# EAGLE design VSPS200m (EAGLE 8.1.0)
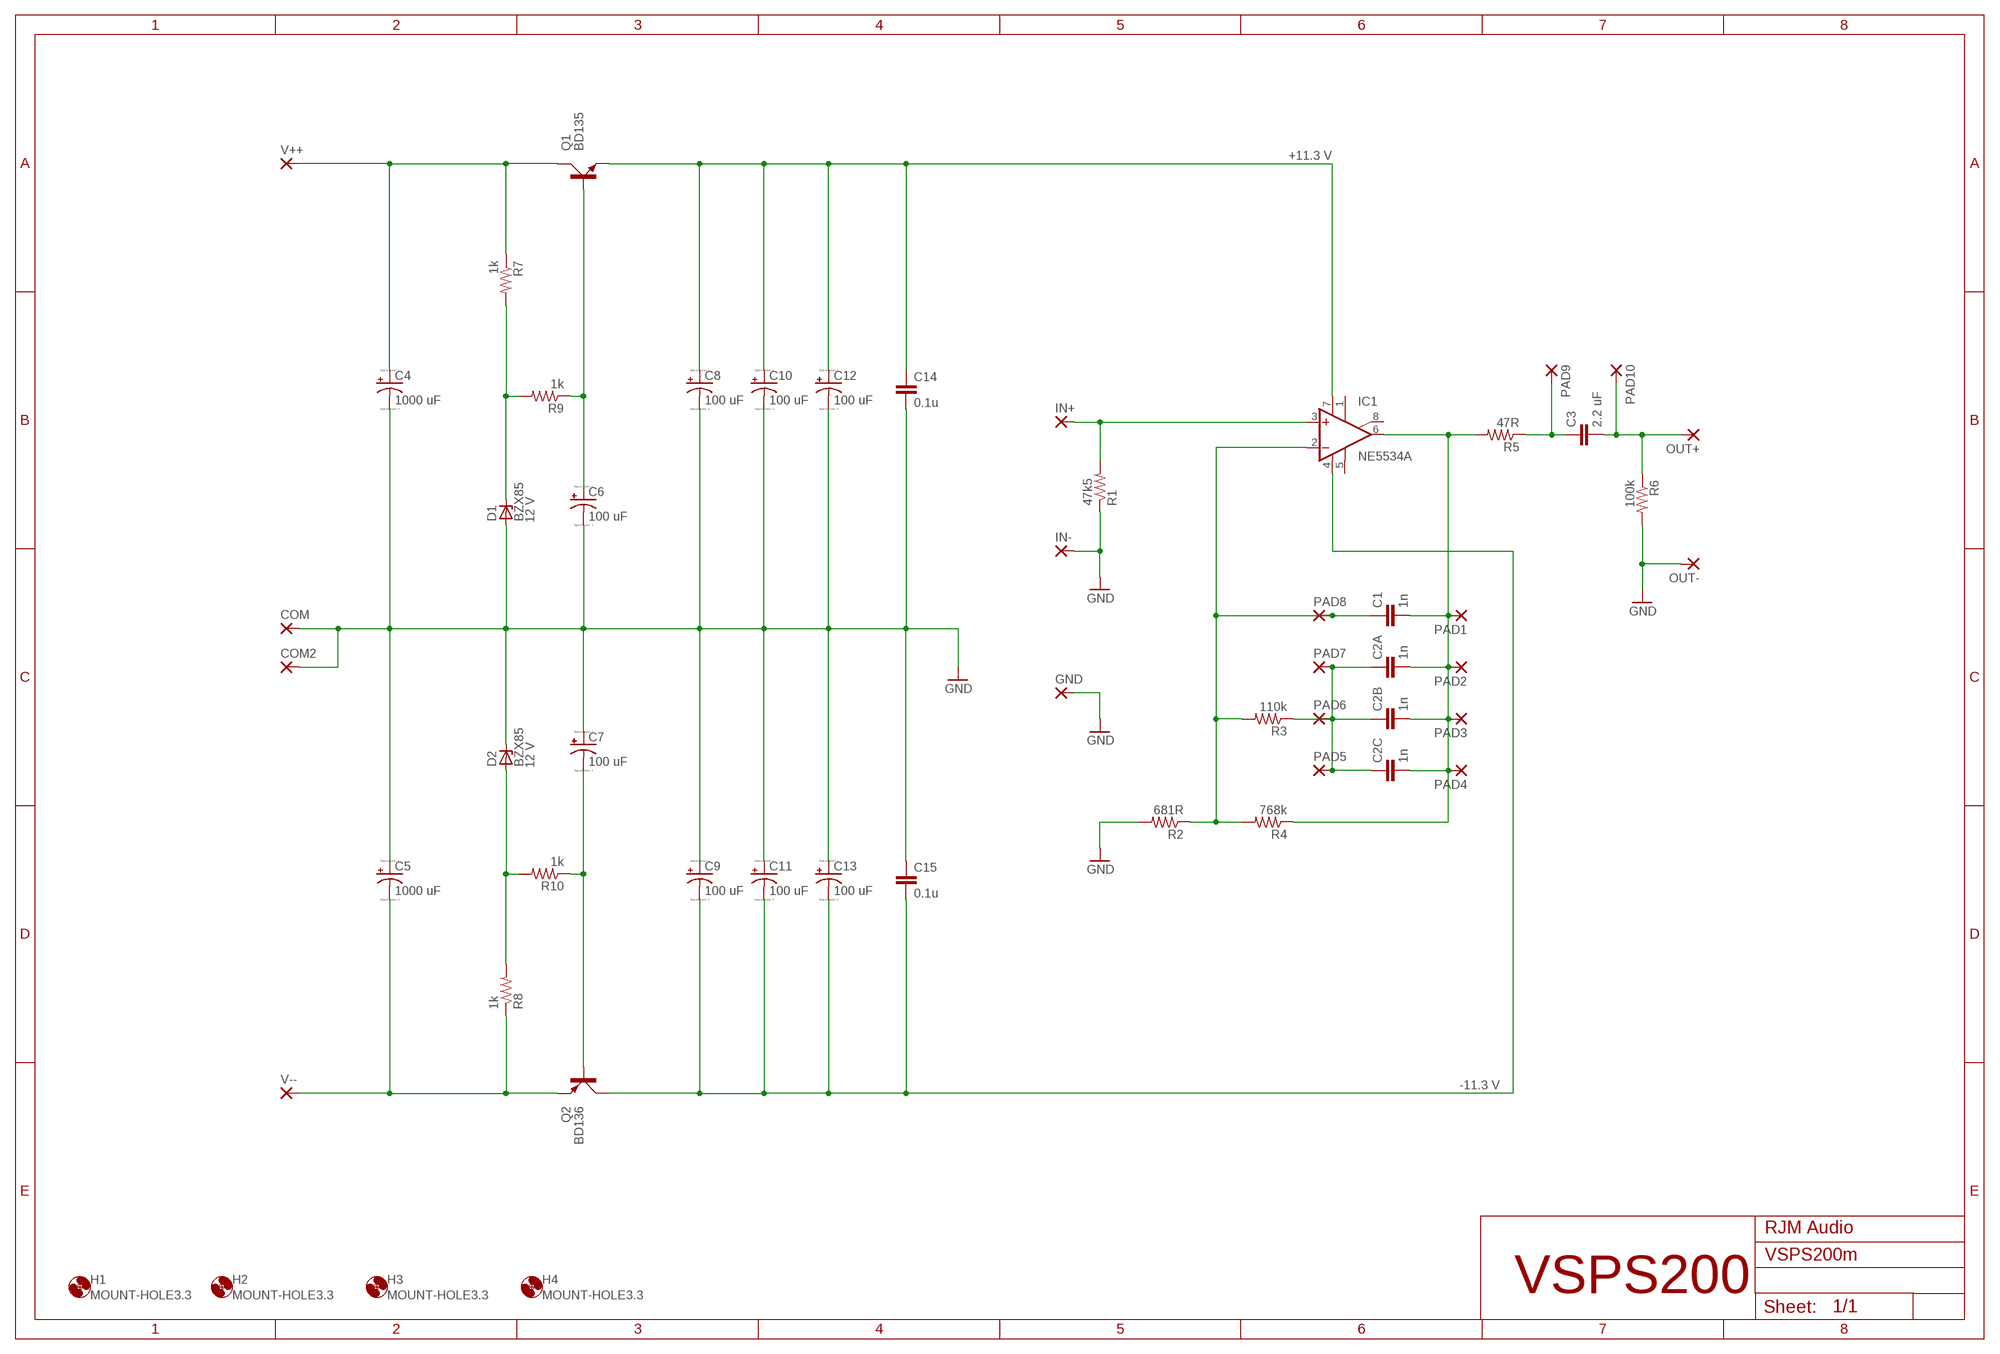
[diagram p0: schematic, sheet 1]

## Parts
C1  1n  C-EU050-045X075  [C050-045X075]
C2A  1n  C-EU050-045X075  [C050-045X075]
C2B  1n  C-EU050-045X075  [C050-045X075]
C2C  1n  C-EU050-045X075  [C050-045X075]
C3  2.2 uF  C-EU375-155X418  [C375-155X418]
C4  1000 uF  CPOL-USE5-10.5  [E5-10,5]
C5  1000 uF  CPOL-USE5-10.5  [E5-10,5]
C6  100 uF  CPOL-USE2.5-6  [E2,5-6]
C7  100 uF  CPOL-USE2.5-6  [E2,5-6]
C8  100 uF  CPOL-USE2.5-6  [E2,5-6]
C9  100 uF  CPOL-USE2.5-6  [E2,5-6]
C10  100 uF  CPOL-USE2.5-6  [E2,5-6]
C11  100 uF  CPOL-USE2.5-6  [E2,5-6]
C12  100 uF  CPOL-USE2.5-6  [E2,5-6]
C13  100 uF  CPOL-USE2.5-6  [E2,5-6]
C14  0.1u  C-EU050-024X044  [C050-024X044]
C15  0.1u  C-EU050-024X044  [C050-024X044]
COM  3,17/1,3  [3,17/1,3]
COM2  3,17/1,3  [3,17/1,3]
D1  BZX85  [DO41Z10]
D2  BZX85  [DO41Z10]
GND  3,17/1,3  [3,17/1,3]
H1  MOUNT-HOLE3.3  [3,3]
H2  MOUNT-HOLE3.3  [3,3]
H3  MOUNT-HOLE3.3  [3,3]
H4  MOUNT-HOLE3.3  [3,3]
IC1  NE5534A  OPA124P  [DIL08]
IN+  3,17/1,3  [3,17/1,3]
IN-  3,17/1,3  [3,17/1,3]
OUT+  3,17/1,3  [3,17/1,3]
OUT-  3,17/1,3  [3,17/1,3]
PAD1  2,15/1,0  [2,15/1,0]
PAD2  2,15/1,0  [2,15/1,0]
PAD3  2,15/1,0  [2,15/1,0]
PAD4  2,15/1,0  [2,15/1,0]
PAD5  2,15/1,0  [2,15/1,0]
PAD6  2,15/1,0  [2,15/1,0]
PAD7  2,15/1,0  [2,15/1,0]
PAD8  2,15/1,0  [2,15/1,0]
PAD9  3,17/1,3  [3,17/1,3]
PAD10  3,17/1,3  [3,17/1,3]
Q1  BD135  BD139  [TO126AV]
Q2  BD136  BD140  [TO126AV]
R1  47k5  R-US_0207/10  [0207/10]
R2  681R  R-US_0207/10  [0207/10]
R3  110k  R-US_0207/10  [0207/10]
R4  768k  R-US_0207/10  [0207/10]
R5  47R  R-US_0207/10  [0207/10]
R6  100k  R-US_0207/10  [0207/10]
R7  1k  R-US_0207/10  [0207/10]
R8  1k  R-US_0207/10  [0207/10]
R9  1k  R-US_0207/10  [0207/10]
R10  1k  R-US_0207/10  [0207/10]
V++  3,17/1,3  [3,17/1,3]
V--  3,17/1,3  [3,17/1,3]

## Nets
GND: C4.- C5.+ C6.- C7.+ C8.- C9.+ C10.- C11.+ C12.- C13.+ C14.2 C15.1 COM2.1(P) COM.1(P) D1.A D2.C GND.1(P) IN-.1(P) OUT-.1(P) R1.1 R2.2 R6.2
N$1: C6.+ Q1.B R9.1
N$2: D1.C R7.2 R9.2
N$3: C7.- Q2.B R10.1
N$4: D2.A R8.2 R10.2
N$5: C2A.1 C2B.1 C2C.1 PAD5.1(P) PAD6.1(P) PAD7.1(P) R3.1
N$6: C1.1 IC1.2(-IN) PAD8.1(P) R2.1 R3.2 R4.2
N$16: C3.1 PAD9.1(P) R5.1
NINV: IC1.3(+IN) IN+.1(P) R1.2
OUT: C1.2 C2A.2 C2B.2 C2C.2 IC1.6(OUT) PAD1.1(P) PAD2.1(P) PAD3.1(P) PAD4.1(P) R4.1 R5.2
OUT+: C3.2 OUT+.1(P) PAD10.1(P) R6.1
V+: C8.+ C10.+ C12.+ C14.1 IC1.7(V+) Q1.E
V++: C4.+ Q1.C R7.1 V++.1(P)
V-: C9.- C11.- C13.- C15.2 IC1.4(V-) Q2.C
V--: C5.- Q2.E R8.1 V--.1(P)
Unconnected: IC1.1(TRIM1) IC1.5(TRIM2) IC1.8(SUBS)

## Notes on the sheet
- +11.3 V
- 12 V
- 12 V
- -11.3 V
- RJM Audio
- VSPS200

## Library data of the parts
C1 C2A C2B C2C C3 = resistor:C-EU: CAPACITOR, European symbol
C4-C13 = resistor:CPOL-US: POLARIZED CAPACITOR, American symbol
C14 C15 = rcl:C-EU: CAPACITOR, European symbol
COM COM2 GND IN+ IN- OUT+ OUT- PAD9 PAD10 V++ V-- = wirepad:3,17/1,3: THROUGH-HOLE PAD
D1 D2 = diode:BZX85: Z DIODE
H1-H4 = holes:MOUNT-HOLE: MOUNTING HOLE with drill center marker
IC1 = burr-brown:OPA124: Difet Operational Amplifier Low Noise, Precision; OC_FARNELL: unknown; OC_NEWARK: unknown
PAD1-PAD8 = wirepad:2,15/1,0: THROUGH-HOLE PAD
Q1 = transistor-power:BD139: NPN TRANSISTOR
Q2 = transistor-power:BD140: PNP TRANSISTOR
R1-R10 = resistor:R-US_: RESISTOR, American symbol

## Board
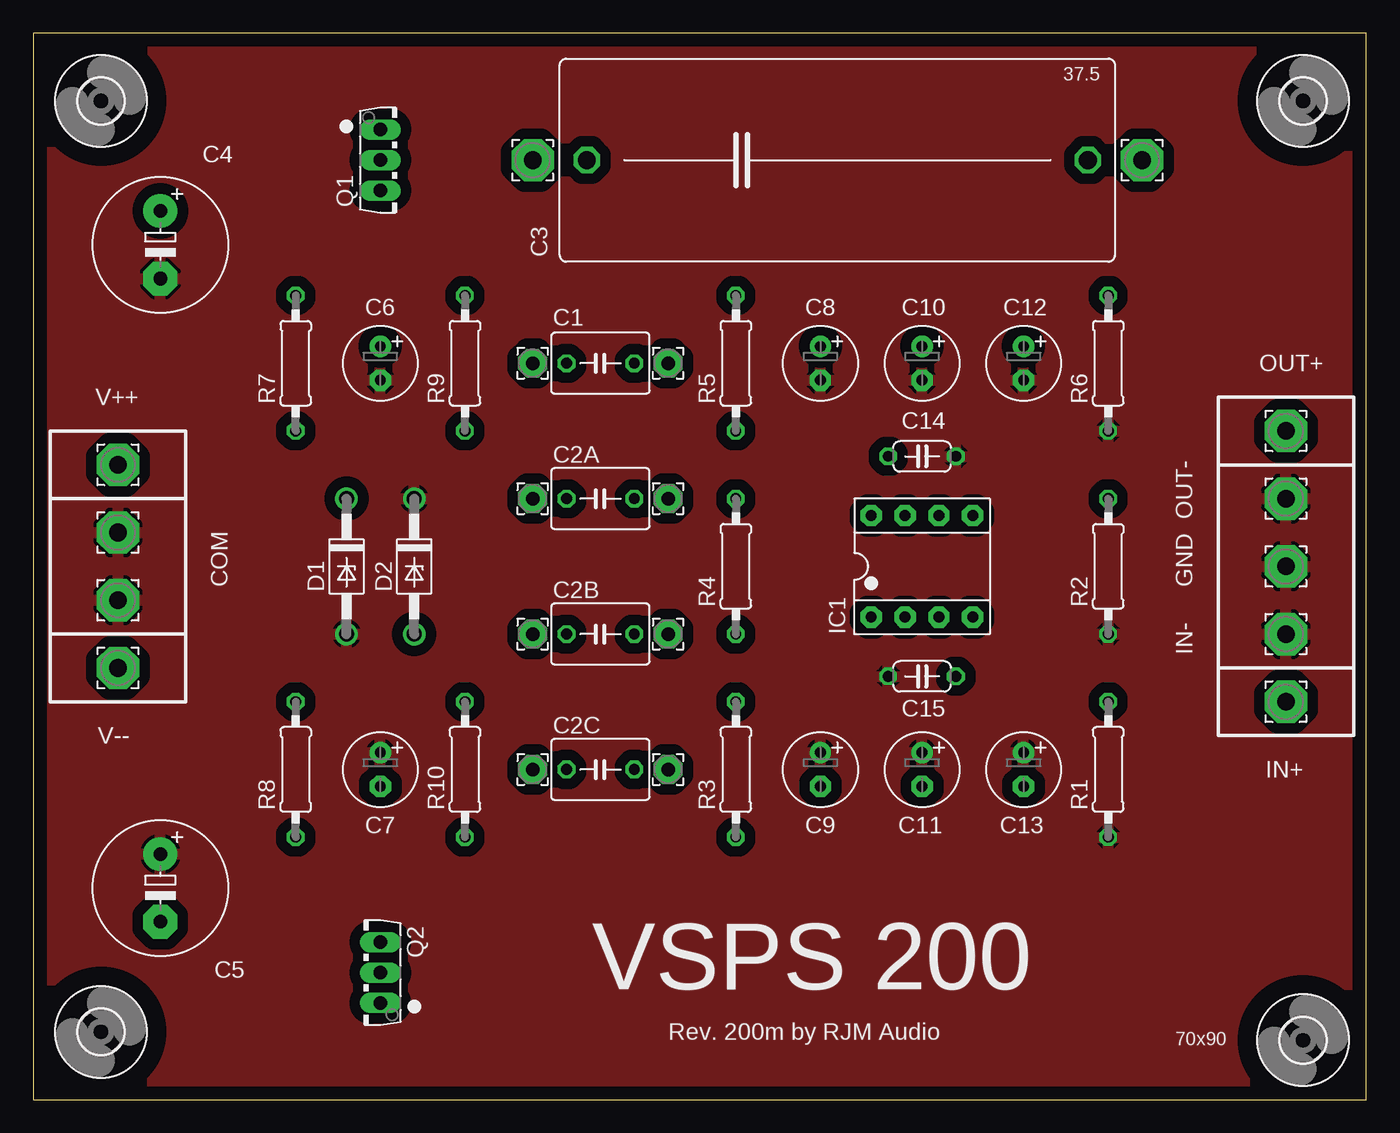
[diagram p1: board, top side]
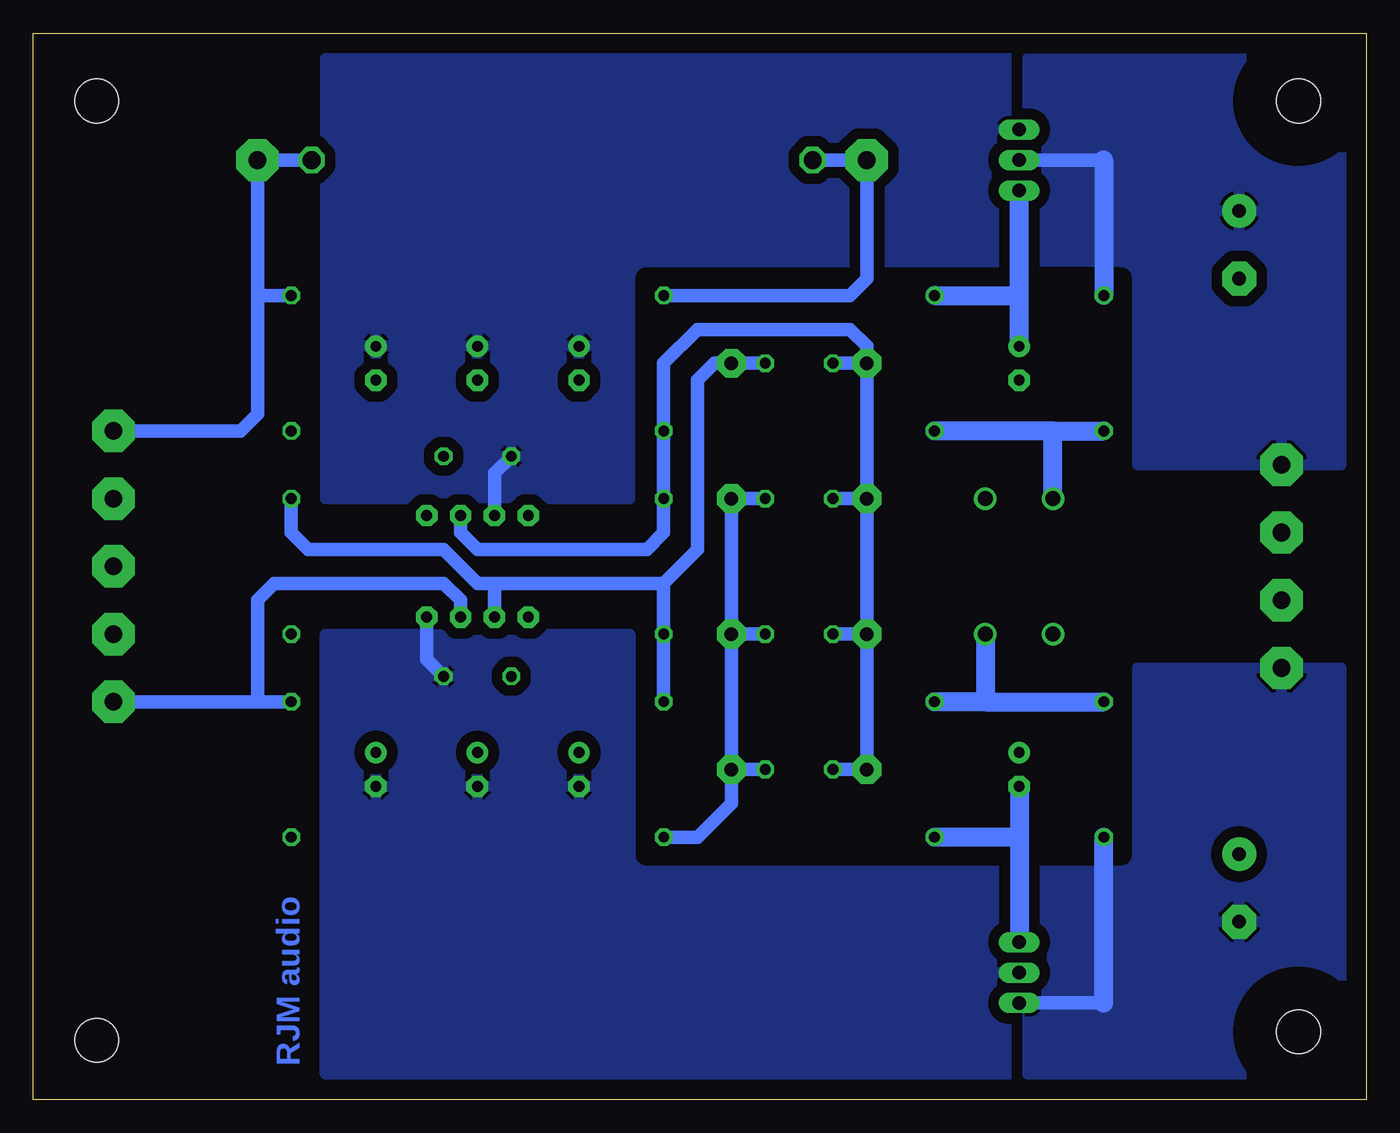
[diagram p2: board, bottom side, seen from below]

Size 100 x 80 mm. Coordinates in mm from the lower left corner, seen from the top.
Outline: 0,0 100,0 100,80 0,80 0,0
Copper layers (1*16): Top 0.035mm / dielectric 1.5mm / Bottom 0.035mm
Design rules "default": minimum track width 10mil, minimum drill 24mil, track to track 8mil, track to pad 8mil, pad to pad 8mil, via to via 8mil, smd to smd 8mil, copper to edge 40mil, drill to drill 8mil, minimum pad ring 10mil, minimum via ring 8mil, stop-mask expansion 4mil, vias tented up to drill 0mil, thermal gap 10mil

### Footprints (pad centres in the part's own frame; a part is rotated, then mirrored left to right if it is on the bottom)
C050-045X075 = drill 0.813 octagon: 1 -2.54,0; 2 2.54,0
C375-155X418 = drill 1.321 octagon: 1 -18.796,0; 2 18.796,0
E5-10,5 = drill 1.016 pad 2.54: + -2.54,0 | drill 1.016 pad 2.54 octagon: - 2.54,0
E2,5-6 = drill 0.813 pad 1.6: + -1.27,0 | drill 0.813 pad 1.6 octagon: - 1.27,0
C050-024X044 = drill 0.813 octagon: 1 -2.54,0; 2 2.54,0
3,17/1,3 = drill 1.321 pad 3.175 octagon: 1 0,0
DO41Z10 = drill 1.118: A 5.08,0; C -5.08,0
3,3 = hole 3.3: 0,0
DIL08 = drill 0.813 pad 1.6 octagon: 1 -3.81,-3.81; 2 -1.27,-3.81; 3 1.27,-3.81; 4 3.81,-3.81; 5 3.81,3.81; 6 1.27,3.81; 7 -1.27,3.81; 8 -3.81,3.81
2,15/1,0 = drill 1.016 pad 2.159 octagon: 1 0,0
TO126AV = drill 1.016 long: B 2.286,-1.27; C 0,-1.27; E -2.286,-1.27
0207/10 = drill 0.813 octagon: 1 -5.08,0; 2 5.08,0

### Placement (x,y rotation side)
C1  42.55,55.25 180 top
C2A  42.55,45.09 180 top
C2B  42.55,34.93 180 top
C2C  42.55,24.76 180 top
C3  60.33,70.48 0 top
C4  9.53,64.13 270 top
C5  9.53,15.88 270 top
C6  26.04,55.25 270 top
C7  26.04,24.76 270 top
C8  59.05,55.25 270 top
C9  59.05,24.76 270 top
C10  66.67,55.25 270 top
C11  66.67,24.76 270 top
C12  74.3,55.25 270 top
C13  74.3,24.76 270 top
C14  66.67,48.26 0 top
C15  66.67,31.75 0 top
COM  6.35,37.47 0 top
COM2  6.35,42.55 0 top
D1  23.49,40.01 270 top
D2  28.57,40.01 270 top
GND  93.98,40.01 0 top
H1  5.08,74.93 0 top
H2  95.25,74.93 0 top
H3  5.08,5.08 0 top
H4  95.25,4.45 0 top
IC1  66.67,40.01 0 top
IN+  93.98,29.84 0 top
IN-  93.98,34.93 0 top
OUT+  93.98,50.16 0 top
OUT-  93.98,45.09 0 top
PAD1  37.47,45.09 270 top
PAD2  37.47,34.93 270 top
PAD3  37.47,24.76 270 top
PAD4  37.47,55.25 270 top
PAD5  47.62,34.93 270 top
PAD6  47.62,24.76 270 top
PAD7  47.62,45.09 270 top
PAD8  47.62,55.25 270 top
PAD9  37.47,70.48 270 top
PAD10  83.18,70.48 270 top
Q1  27.3,70.48 270 top
Q2  24.76,9.53 90 top
R1  80.64,24.76 90 top
R2  80.64,40.01 270 top
R3  52.71,24.76 90 top
R4  52.71,40.01 270 top
R5  52.71,55.25 270 top
R6  80.64,55.25 270 top
R7  19.68,55.25 270 top
R8  19.68,24.76 90 top
R9  32.39,55.25 270 top
R10  32.39,24.76 90 top
V++  6.35,47.62 0 top
V--  6.35,32.39 0 top

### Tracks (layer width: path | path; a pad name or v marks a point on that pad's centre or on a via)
GND
  pour Top (isolate 0.813): -1.27,81.28 101.6,81.28 101.6,-1.27 -1.27,-1.27
N$1
  Bottom 1.422: 26.04,60.33 Q1.B | R9.1 26.04,60.33 | C6.+ 26.04,60.33
N$2
  Bottom 1.422: 23.49,50.16 R9.2 | D1.C 23.49,50.16 | 23.49,50.16 R7.2
N$3
  Bottom 1.422: 26.04,19.68 R10.1 | 26.04,19.68 Q2.B | C7.- 26.04,19.68
N$4
  Bottom 1.422: 28.57,29.84 R8.2 | D2.A 28.57,29.84 | 28.57,29.84 R10.2
N$5
  Bottom 1.016: PAD6.1 C2C.1 | C2B.1 PAD5.1 | C2A.1 PAD7.1 PAD5.1 | R3.1 50.16,19.68 47.62,22.22 PAD6.1 | PAD5.1 PAD6.1
N$6
  Bottom 1.016: 65.41,38.73 IC1.2 | 52.71,38.73 65.41,38.73 | 52.71,38.73 R4.2 R3.2 | R2.1 80.64,42.55 79.38,41.27 76.83,41.27 69.21,41.27 66.67,38.73 65.41,38.73 | 52.71,38.73 50.16,41.27 50.16,53.98 48.9,55.25 PAD8.1 C1.1
N$16
  Bottom 1.016: C3.1 PAD9.1 37.47,61.59 38.73,60.33 R5.1
NINV
  Bottom 1.016: IC1.3 67.94,37.47 69.21,38.73 81.91,38.73 83.18,37.47 83.18,29.84 | 83.18,29.84 R1.2 | IN+.1 83.18,29.84
OUT
  Bottom 1.016: C1.2 PAD4.1 | C2C.2 PAD3.1 PAD2.1 | C2B.2 PAD2.1 | C2A.2 PAD1.1 | IC1.6 67.94,42.55 66.67,41.27 53.98,41.27 52.71,42.55 R4.1 R5.2 52.71,55.25 50.16,57.79 38.73,57.79 37.47,56.52 PAD4.1 | PAD2.1 PAD1.1 | PAD1.1 PAD4.1
OUT+
  Bottom 1.016: C3.2 PAD10.1 83.18,60.33 | 83.18,60.33 83.18,51.44 84.45,50.16 OUT+.1 | R6.1 83.18,60.33
V+
  Bottom 1.016: IC1.7 65.41,46.99 C14.1
  pour Bottom (isolate 0.813, rank 3): 26.67,62.87 26.67,78.1 78.1,78.1 78.1,45.09 55.25,45.09 55.25,61.59 arc90 53.98,62.87
V++
  Bottom 1.016: Q1.C 19.68,70.48
  Bottom 1.422: 19.68,70.48 R7.1
  pour Bottom (isolate 0.813, rank 2): 1.91,78.1 1.91,47.62 17.14,47.62 17.14,61.59 arc-90 18.41,62.87 25.4,62.87 25.4,78.1
V-
  Bottom 1.016: IC1.4 70.48,33.02 C15.2
  pour Bottom (isolate 0.813, rank 3): 26.67,17.14 26.67,1.91 78.1,1.91 78.1,34.93 55.25,34.93 55.25,18.41 arc-90 53.98,17.14
V--
  Bottom 1.016: Q2.E 19.68,7.24
  Bottom 1.422: 19.68,7.24 R8.1
  pour Bottom (isolate 0.813, rank 2): 1.91,32.39 1.91,1.91 25.4,1.91 25.4,17.14 18.41,17.14 arc-90 17.14,18.41 17.14,32.39

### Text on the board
Bottom: RJM audio
tPlace: 37.5 | VSPS 200 | 70x90 | Rev. 200m by RJM Audio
